{attribute 'no-analysis'}
FUNCTION_BLOCK FB_SboControlEnhanced EXTENDS FB_SboControl
VAR
END_VAR

METHOD Execute : BOOL
VAR
	bTestOk: BOOL; (*Used to cache the return value of the last '_OperativeTest' or '_DynamicTest' method call*)
	eError: E_AcsiServiceError; (*Used to cache the returned error of the last '_OperativeTest' or '_DynamicTest' method call*)
	tValue: T_UtcTime; (*Used to cache the current system time for 'tOpOk'*)
END_VAR
IF (_ipCtrl <> 0) AND_THEN (_ipCtrl.ipOper <> 0) THEN
	(* Initialize function block in the first cycle *)
	IF NOT bInit THEN
		_Init();
		bInit:=TRUE;
	END_IF

	CASE _eControlState OF
		E_SboControlState.Unselected:
			(* Check if ControlState changed in the last cycle *)
			IF bNewState THEN
				bNewState:=FALSE;
				_Reset();
			END_IF
			(* Check if a valid Cancel_req was received *)
			IF bCancelReq THEN
				bCancelReq:=FALSE;
			END_IF
			(* Check if a valid SelVal_req was received *)
			IF bSelValReq THEN
				bSelValReq:=FALSE;
				(* Go to next ControlState *)
				_eControlState:=E_SboControlState.Select_PerformTest;
				bNewState:=TRUE;
			END_IF

		E_SboControlState.Select_PerformTest:
			(* Check if ControlState changed in the last cycle *)
			IF bNewState THEN
				bNewState:=FALSE;
			END_IF
			(* Trigger the test until it is finished *)
			IF _Test(bTestOk=>bTestOk, eError=>eError) THEN
				IF bTestOk THEN
					(* Go to next ControlState *)
					_eControlState:=E_SboControlState.WaitForSelection;
				ELSE
					fbSelValCompletion.SetCompleted();
					fbSelValCompletion.eServiceError:=eError;
					(* Go back to ControlState 'Unselected' *)
					_eControlState:=E_SboControlState.Unselected;
				END_IF
				bNewState:=TRUE;
			END_IF

		E_SboControlState.WaitForSelection:
			(* Check if ControlState changed in the last cycle *)
			IF bNewState THEN
				bNewState:=FALSE;
			END_IF
			(* Set 'stSeld' *)
			IF (_ipCtrl.ipStSeld <> 0) THEN
				_ipCtrl.ipStSeld.bValue:=TRUE;
			END_IF
			fbSelValCompletion.SetCompleted();
			(* Go to next ControlState *)
			_eControlState:=E_SboControlState.Ready;
			bNewState:=TRUE;

		E_SboControlState.Ready:
			(* Check if ControlState changed in the last cycle *)
			IF bNewState THEN
				bNewState:=FALSE;
				(* Start timer *)
				IF (_ipCtrl.ipSboTimeout <> 0) THEN
					_fbSboTimer(IN:=TRUE, PT:=DWORD_TO_TIME(_ipCtrl.ipSboTimeout.nValue));
				END_IF
			END_IF
			_fbSboTimer();
			(* Check if a valid Cancel_req was received, 'sboTimeout' was exceeded or the association was lost *)
			IF bCancelReq OR_ELSE _fbSboTimer.Q OR_ELSE ((_ipCurrentAA <> 0) AND_THEN (_ipCurrentAA.eState <> E_AsyncEnvironmentState.Established)) THEN
				bCancelReq:=FALSE;
				_fbSboTimer(IN:=FALSE);
				(* Go to next ControlState *)
				_eControlState:=E_SboControlState.EndSelection;
				bNewState:=TRUE;
			END_IF
			(* Check if a valid Oper_req was received *)
			IF bOperReq THEN
				bOperReq:=FALSE;
				(* Go to next ControlState *)
				_eControlState:=E_SboControlState.PerformTest;
				bNewState:=TRUE;
			END_IF

		E_SboControlState.PerformTest:
			(* Check if ControlState changed in the last cycle *)
			IF bNewState THEN
				bNewState:=FALSE;
				(* Set 'opRcvd' *)
				IF (_ipCtrl.ipOpRcvd <> 0) THEN
					_ipCtrl.ipOpRcvd.bValue:=TRUE;
				END_IF
			END_IF
			(* Check if a valid Cancel_req was received *)
			IF bCancelReq THEN
				bCancelReq:=FALSE;
				(* Send Oper_resp- *)
				_SendLastApplError(ipAA:=_ipCurrentAA, ipCtrlData:=_ipCtrl.ipOper, eError:=E_AcsiApplError.NoError, ipOrigin:=_ipCtrl.ipOper.ipOrigin, ipCtlNum:=_ipCtrl.ipOper.ipCtlNum, eAddCause:=E_AcsiApplAddCause.AbortionByCancel);
				fbOperCompletion.SetCompleted();
				fbOperCompletion.eServiceError:=E_AcsiServiceError.AccessViolation;
				(* Go to ControlState 'EndSelection' *)
				_eControlState:=E_SboControlState.EndSelection;
				bNewState:=TRUE;
			END_IF
			(* Trigger the operative test until it is finished *)
			IF _OperativeTest(bOperativeTestOk=>bTestOk, eError=>eError) THEN
				(* Reset 'opRcvd' *)
				IF (_ipCtrl.ipOpRcvd <> 0) THEN
					_ipCtrl.ipOpRcvd.bValue:=FALSE;
				END_IF
				IF bTestOk THEN
					(* Go to next ControlState *)
					_eControlState:=E_SboControlState.WaitForExecution;
				ELSE
					fbOperCompletion.SetCompleted();
					fbOperCompletion.eServiceError:=eError;
					(* Go to ControlState 'EndSelection' *)
					_eControlState:=E_SboControlState.EndSelection;
				END_IF
				bNewState:=TRUE;
			END_IF

		E_SboControlState.WaitForExecution:
			(* Check if ControlState changed in the last cycle *)
			IF bNewState THEN
				bNewState:=FALSE;
			END_IF
			(* Check if a Cancel_req was received *)
			IF bCancelReq THEN
				bCancelReq:=FALSE;
				(* Send Oper_resp- *)
				_SendLastApplError(ipAA:=_ipCurrentAA, ipCtrlData:=_ipCtrl.ipOper, eError:=E_AcsiApplError.NoError, ipOrigin:=_ipCtrl.ipOper.ipOrigin, ipCtlNum:=_ipCtrl.ipOper.ipCtlNum, eAddCause:=E_AcsiApplAddCause.AbortionByCancel);
				fbOperCompletion.SetCompleted();
				fbOperCompletion.eServiceError:=E_AcsiServiceError.AccessViolation;
				(* Go to ControlState 'EndSelection' *)
				_eControlState:=E_SboControlState.EndSelection;
				bNewState:=TRUE;
			END_IF
			(* Trigger the dynamic test until it is finished *)
			IF _DynamicTest(bDynamicTestOk=>bTestOk, eError=>eError) THEN
				fbOperCompletion.SetCompleted();
				IF bTestOk THEN
					(* Go to next ControlState *)
					IF (_ipBehVal <> 0) AND_THEN ((_ipBehVal.eValue = E_AcsiBeh.TestBlocked) OR_ELSE (_ipBehVal.eValue = E_AcsiBeh.OnBlocked)) THEN
						_eControlState:=E_SboControlState.MirrorBlockedCommand;
					ELSE
						_eControlState:=E_SboControlState.WaitForChange;
					END_IF
				ELSE
					fbOperCompletion.eServiceError:=eError;
					(* Go to ControlState 'EndSelection' *)
					_eControlState:=E_SboControlState.EndSelection;
				END_IF
				bNewState:=TRUE;
			END_IF

		E_SboControlState.WaitForChange:
			(* Check if ControlState changed in the last cycle *)
			IF bNewState THEN
				bNewState:=FALSE;
				(* Set 'opOk' *)
				IF (_ipCtrl.ipOpOk <> 0) THEN
					_ipCtrl.ipOpOk.bValue:=TRUE;
				END_IF
				(* Set 'tOpOk' *)
				IF (_ipCtrl.ipTOpOk <> 0) AND_THEN (_ipCurrentAA <> 0) AND_THEN (_ipCurrentAA.GetSystemTime(tT=>tValue)) THEN
					_ipCtrl.ipTOpOk.tValue:=tValue;
				END_IF
			END_IF
			(* Update value *)
			_SetValue(uCtlVal:=_ipCtrl.ipOper.uCtlVal, ipCtlVal_AV:=_ipCtrl.ipOper.ipCtlVal_AnalogueValue);
			(* Update Timestamp 't' *)
			_UpdateTimestampValue(ipAA:=_ipCurrentAA);

			(* Reset 'opOk' *)
			IF (_ipCtrl.ipOpOk <> 0) THEN
				_ipCtrl.ipOpOk.bValue:=FALSE;
			END_IF
			(* Send CmdTerm_req+ *)
			_SendCommandTerminationReqPos(ipAA:=_ipCurrentAA, ipCtrlData:=_ipCtrl.ipOper);
			(* Go to next ControlState *)
			IF (_ipCtrl.ipSboClass <> 0) AND_THEN (_ipCtrl.ipSboClass.eValue = E_AcsiSboClasses.OperateMany) THEN
				_eControlState:=E_SboControlState.Ready;
			ELSE
				_eControlState:=E_SboControlState.EndSelection;
			END_IF
			bNewState:=TRUE;

		E_SboControlState.MirrorBlockedCommand:
			(* Check if ControlState changed in the last cycle *)
			IF bNewState THEN
				bNewState:=FALSE;
				(* Set 'opOk' *)
				IF (_ipCtrl.ipOpOk <> 0) THEN
					_ipCtrl.ipOpOk.bValue:=TRUE;
				END_IF
				(* Set 'tOpOk' *)
				IF (_ipCtrl.ipTOpOk <> 0) AND_THEN (_ipCurrentAA <> 0) AND_THEN (_ipCurrentAA.GetSystemTime(tT=>tValue)) THEN
					_ipCtrl.ipTOpOk.tValue:=tValue;
				END_IF
			END_IF
			(* Reset 'opOk' *)
			IF (_ipCtrl.ipOpOk <> 0) THEN
				_ipCtrl.ipOpOk.bValue:=FALSE;
			END_IF
			(* Send CmdTerm_req- *)
			_SendCommandTerminationReqNeg(ipAA:=_ipCurrentAA, ipCtrlData:=_ipCtrl.ipOper, eError:=E_AcsiApplError.NoError, ipOrigin:=_ipCtrl.ipOper.ipOrigin, ipCtlNum:=_ipCtrl.ipOper.ipCtlNum, eAddCause:=E_AcsiApplAddCause.BlockedByMode);
			(* Go to next ControlState *)
			IF (_ipCtrl.ipSboClass <> 0) AND_THEN (_ipCtrl.ipSboClass.eValue = E_AcsiSboClasses.OperateMany) THEN
				_eControlState:=E_SboControlState.Ready;
			ELSE
				_eControlState:=E_SboControlState.EndSelection;
			END_IF
			bNewState:=TRUE;

		E_SboControlState.EndSelection:
			(* Check if ControlState changed in the last cycle *)
			IF bNewState THEN
				bNewState:=FALSE;
				(* Reset 'stSeld' *)
				IF (_ipCtrl.ipStSeld <> 0) THEN
					_ipCtrl.ipStSeld.bValue:=FALSE;
				END_IF
			END_IF
			(* Go to next ControlState *)
			_eControlState:=E_SboControlState.Unselected;
			bNewState:=TRUE;
	END_CASE
END_IF

(* Monitor transmission of LastApplError *)
CASE _nLastApplErrorReqState OF
	0:	;
	1:
		IF (_ipLastApplErrorReq <> 0) THEN
			Execute:=_ipLastApplErrorReq.Execute();
			IF NOT _ipLastApplErrorReq.IsBusy() THEN
				IF _ipLastApplErrorReq.IsCompleted() THEN
					SUPER^.SetCompleted();
				ELSE
					SUPER^.CopyFrom(ipSource:=_ipLastApplErrorReq);
				END_IF
				_nLastApplErrorReqState:=0;
			END_IF
		END_IF
END_CASE
(* Monitor transmission of CommandTermination *)
CASE _nCmdTermReqState OF
	0:	RETURN;
	1:
		IF (_ipCmdTermReq <> 0) THEN
			Execute:=_ipCmdTermReq.Execute();
			IF NOT _ipCmdTermReq.IsBusy() THEN
				IF _ipCmdTermReq.IsCompleted() THEN
					SUPER^.SetCompleted();
				ELSE
					SUPER^.CopyFrom(ipSource:=_ipLastApplErrorReq);
				END_IF
				_nCmdTermReqState:=0;
			END_IF
		END_IF
END_CASE
END_METHOD

METHOD OnCompletionWaitEvent : BOOL
VAR_INPUT
	ipDai: I_AcsiDataAccessInfoClass;
	ipData: I_AcsiCommonDataClass;
	eFc: E_AcsiFc;
END_VAR
VAR_OUTPUT
	ipResult: I_AcsiServiceResultClass := fbCompletion;
END_VAR
VAR
	eServiceError: E_AcsiServiceError;
	ipAA: I_ScsmAssociationClass; (*Interface pointer to application association*)
END_VAR
fbCompletion.SetCompleted();
IF (ipDai = 0) OR_ELSE (ipData = 0) THEN
	fbCompletion.eServiceError:=E_AcsiServiceError.AccessViolation;
	RETURN;
END_IF

(* Check if an Operate request is received *)
IF (ipDai.eService = E_AcsiServiceType.SetDataValues) THEN
	IF	(ipData.sObjectName = 'Oper') THEN
		fbOperCompletion.SetBusy();
		ipResult:=fbOperCompletion;
		bOperReq:=TRUE;
		OnCompletionWaitEvent:=TRUE;
	ELSIF (ipData.sObjectName = 'SBOw') THEN
		ScsmAssociation_From_Dai(in:=ipDai, out=>_ipCurrentAA);
		fbSelValCompletion.SetBusy();
		ipResult:=fbSelValCompletion;
		bSelValReq:=TRUE;
		OnCompletionWaitEvent:=TRUE;
	ELSIF (ipData.sObjectName = 'Cancel') THEN
		fbCancelCompletion.SetCompleted();
		ipResult:=fbCancelCompletion;
		IF _CheckCancelReq(ipDai:=ipDai, eError=>eServiceError) THEN
			bCancelReq:=TRUE;
		ELSE
			fbCancelCompletion.eServiceError:=eServiceError;
		END_IF
	END_IF
END_IF
END_METHOD

(*Implementation of user application data update event method.*)
METHOD OnGetVEvent
VAR_INPUT
	ipDai: I_AcsiDataAccessInfoClass; (*Additional data access info*)
	ipData: I_AcsiCommonDataClass; (*Interface pointer to data object*)
	eFc: E_AcsiFc; (*Functional constraint*)
END_VAR
VAR
END_VAR
END_METHOD

(*Implementation of user application data update event method.*)
METHOD OnGetVPreEvent : E_AcsiServiceError
VAR_INPUT
	ipDai: I_AcsiDataAccessInfoClass; (*Additional data access info*)
	ipData: I_AcsiCommonDataClass; (*Interface pointer to data object*)
	eFc: E_AcsiFc; (*Functional constraint*)
END_VAR
VAR
END_VAR
END_METHOD

(*Implementation of user application data update event method.*)
METHOD OnSetVPreEvent : E_AcsiServiceError
VAR_INPUT
	ipDai: I_AcsiDataAccessInfoClass; (*Additional data access info*)
	ipMemory: I_AnyMemoryBuffer; (*Interface pointer to buffer containig new value data*)
	ipData: I_AcsiCommonDataClass; (*Interface pointer to data object*)
	eFc: E_AcsiFc; (*Functional constraint*)
END_VAR
VAR_OUTPUT
	ipLastApplError: I_AcsiDATypeLastApplError; (*IF <> 0 => send LastApplError request*)
END_VAR
VAR
	ipAA: I_ScsmAssociationClass; (*Interface pointer to application association*)
	bItself: BOOL; (*If TRUE => Checking object is sub-data object itself*)
END_VAR
IF (eFc = E_AcsiFc.CO) AND_THEN (_ipCtrl <> 0) AND_THEN (ipDai <> 0) AND_THEN (ipDai.Write) AND_THEN (ipDai.ipAccessData <> 0) AND_THEN (ipData <> 0)
AND_THEN ScsmAssociation_From_Dai(in:=ipDai, out=>ipAA) THEN
	IF (_ipCtrl.ipOper <> 0) AND_THEN (_ipCtrl.ipOper.ipOrigin <> 0) AND_THEN (_ipCtrl.ipOper.ipCtlNum <> 0) THEN
		(* Check for invalid write attemps to prevent 'Oper' from being overwritten while a control request is being executed *)
		IF (ipDai.ipAccessData.sObjectName = 'Oper') THEN
			(* Only allow 'Oper' requests in state 'Ready' *)
			IF (_eControlState <> E_SboControlState.Ready) THEN
				ipLastApplError:=ipAA.SetAdditionalCauseDiag(ipCtrlData:=_ipCtrl.ipOper, eError:=E_AcsiApplError.NoError, stOrigin:=_ipCtrl.ipOper.ipOrigin.stOrigin, nCtlNum:=_ipCtrl.ipOper.ipCtlNum.nValue, eAddCause:=E_AcsiApplAddCause.CommandAlreadyInExecution);
				OnSetVPreEvent:=E_AcsiServiceError.AccessViolation;
				RETURN;
			END_IF
		ELSIF (_ipCtrl.ipOper.HasDataSubObject(ipData:=ipDai.ipAccessData, bItself=>bItself) AND_THEN (NOT bItself)) THEN
			(* Don't allow write access to subdata of 'Oper'*)
			ipLastApplError:=ipAA.SetAdditionalCauseDiag(ipCtrlData:=_ipCtrl.ipOper, eError:=E_AcsiApplError.NoError, stOrigin:=_ipCtrl.ipOper.ipOrigin.stOrigin, nCtlNum:=_ipCtrl.ipOper.ipCtlNum.nValue, eAddCause:=E_AcsiApplAddCause.NotSupported);
			OnSetVPreEvent:=E_AcsiServiceError.AccessViolation;
			RETURN;
		END_IF
	END_IF
	IF (_ipCtrl.ipSBOw <> 0) AND_THEN (_ipCtrl.ipSBOw.ipOrigin <> 0) AND_THEN (_ipCtrl.ipSBOw.ipCtlNum <> 0) THEN
		(* Check for invalid write attemps to prevent 'SBOw' from being overwritten while a control request is being executed *)
		IF (ipDai.ipAccessData.sObjectName = 'SBOw') THEN
			(* Only allow 'SelectWithValue' requests in state 'Unselected' *)
			IF (_eControlState <> E_SboControlState.Unselected) THEN
				ipLastApplError:=ipAA.SetAdditionalCauseDiag(ipCtrlData:=_ipCtrl.ipSBOw, eError:=E_AcsiApplError.NoError, stOrigin:=_ipCtrl.ipSBOw.ipOrigin.stOrigin, nCtlNum:=_ipCtrl.ipSBOw.ipCtlNum.nValue, eAddCause:=E_AcsiApplAddCause.CommandAlreadyInExecution);
				OnSetVPreEvent:=E_AcsiServiceError.AccessViolation;
				RETURN;
			ELSIF (_ipCtrl.ipSBOw.HasDataSubObject(ipData:=ipDai.ipAccessData, bItself=>bItself) AND_THEN (NOT bItself)) THEN
				(* Don't allow write access to subdata of 'SBOw'*)
				ipLastApplError:=ipAA.SetAdditionalCauseDiag(ipCtrlData:=_ipCtrl.ipSBOw, eError:=E_AcsiApplError.NoError, stOrigin:=_ipCtrl.ipSBOw.ipOrigin.stOrigin, nCtlNum:=_ipCtrl.ipSBOw.ipCtlNum.nValue, eAddCause:=E_AcsiApplAddCause.NotSupported);
				OnSetVPreEvent:=E_AcsiServiceError.AccessViolation;
				RETURN;
			END_IF
		END_IF
	END_IF
	IF (_ipCtrl.ipCancel <> 0) AND_THEN (_ipCtrl.ipCancel.ipOrigin <> 0) AND_THEN (_ipCtrl.ipCancel.ipCtlNum <> 0) THEN
		IF (ipDai.ipAccessData.sObjectName <> 'Cancel') AND_THEN (_ipCtrl.ipCancel.HasDataSubObject(ipData:=ipDai.ipAccessData)) THEN
			(* Don't allow write access to subdata of 'Cancel'*)
			ipLastApplError:=ipAA.SetAdditionalCauseDiag(ipCtrlData:=_ipCtrl.ipCancel, eError:=E_AcsiApplError.NoError, stOrigin:=_ipCtrl.ipCancel.ipOrigin.stOrigin, nCtlNum:=_ipCtrl.ipCancel.ipCtlNum.nValue, eAddCause:=E_AcsiApplAddCause.NotSupported);
			OnSetVPreEvent:=E_AcsiServiceError.AccessViolation;
			RETURN;
		END_IF
	END_IF
END_IF
END_METHOD

END_FUNCTION_BLOCK
